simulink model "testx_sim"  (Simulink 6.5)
settings: Solver=ode45  StartTime=0.0  StopTime=300.0  RelTol=1e-3
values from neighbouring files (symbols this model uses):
  A = [ -0.195 0.195; 0.195 -0.205]    [testx.m]    (also in podklad.m = [dh1_h10 dh1_h20 0; kockaLQG.m = [0 1 0 0 0; kockaLQR.m = [0 1 0 0 0; kulicka_na_tyci_LQG_podklad.m = [0 0;1 0])
  B = [0.0047; 0]    [testx.m]    (also in podklad.m = [dh1_q0; kockaLQG.m = [0; kockaLQR.m = [0; kulicka_na_tyci_LQG_podklad.m = [7.14;0])
  C = [0 1]    [testx.m]    (also in podklad.m = [0 0 1]; kockaLQG.m = [1 0 0 0 0]; kockaLQR.m = [1 0 0 0 0]; kulicka_na_tyci_LQG_podklad.m)
  D = [0]    [testx.m]    (also in podklad.m = 0; kockaLQG.m; kockaLQR.m; kulicka_na_tyci_LQG_podklad.m = 0)
  K = tf(num,den)    [phinf2.m]
  Ng = Nu + K*Nx    [lqr_kompenzace.m]    (also in testx.m = lqr_kompenzace(A,B,C,D,K); kockaLQG.m = lqr_kompenzace(A,B,C,D,K); kockaLQR.m = lqr_kompenzace(A,B,C,D,K); kulicka_na_tyci_LQG_podklad.m = lqr_kompenzace(A,B,C,D,K))
undefined symbols (not defined in the file or in its folder): KA, KB, KC, KD, L
libraries: simulink_extras x2

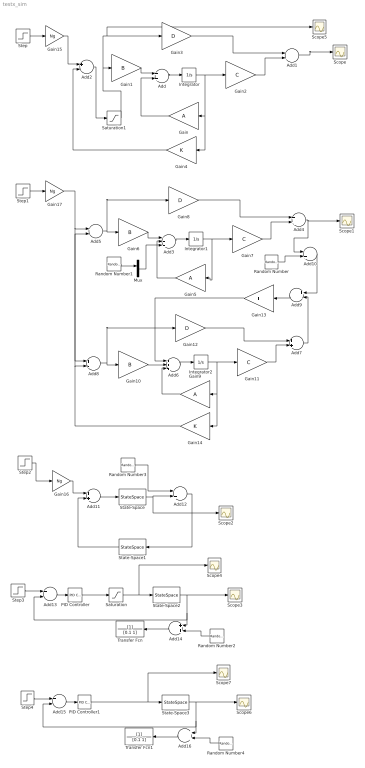
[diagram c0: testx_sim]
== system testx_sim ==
  Add{,1,4,7,10..12} (7 alike) : Sum  OutScaling=2^-10
  Add{2,5,8,13,15} (5 alike) : Sum  Inputs=+-  OutScaling=2^-10
  Add14 : Sum  Orientation=left  OutScaling=2^-10
  Add16 : Sum  Orientation=left  OutScaling=2^-10
  Add3 : Sum  Inputs=+++  OutScaling=2^-10
  Add6 : Sum  Inputs=+++  OutScaling=2^-10
  Add9 : Sum  Orientation=left  Inputs=+-  OutScaling=2^-10
  Gain : Gain  Orientation=left  Gain=A  Multiplication=Matrix(K*u) (u vector)
  Gain1 : Gain  Gain=B  Multiplication=Matrix(K*u) (u vector)
  Gain10 : Gain  Gain=B  Multiplication=Matrix(K*u) (u vector)
  Gain11 : Gain  Gain=C  Multiplication=Matrix(K*u) (u vector)
  Gain12 : Gain  Gain=D  Multiplication=Matrix(K*u) (u vector)
  Gain13 : Gain  Orientation=left  Gain=L  Multiplication=Matrix(K*u) (u vector)
  Gain14 : Gain  Orientation=left  Gain=K  Multiplication=Matrix(K*u) (u vector)
  Gain15 : Gain  Gain=Ng
  Gain16 : Gain  Gain=Ng
  Gain17 : Gain  Gain=Ng
  Gain2 : Gain  Gain=C  Multiplication=Matrix(K*u) (u vector)
  Gain3 : Gain  Gain=D  Multiplication=Matrix(K*u) (u vector)
  Gain4 : Gain  Orientation=left  Gain=K  Multiplication=Matrix(K*u) (u vector)
  Gain5 : Gain  Orientation=left  Gain=A  Multiplication=Matrix(K*u) (u vector)
  Gain6 : Gain  Gain=B  Multiplication=Matrix(K*u) (u vector)
  Gain7 : Gain  Gain=C  Multiplication=Matrix(K*u) (u vector)
  Gain8 : Gain  Gain=D  Multiplication=Matrix(K*u) (u vector)
  Gain9 : Gain  Orientation=left  Gain=A  Multiplication=Matrix(K*u) (u vector)
  Integrator : Integrator
  Integrator1 : Integrator
  Integrator2 : Integrator
  Mux : Mux  Inputs=2
  PID Controller : simulink_extras/Additional Linear/PID Controller  SystemSampleTime=-1  P=50  I=0.1  D=7
  PID Controller1 : simulink_extras/Additional Linear/PID Controller  SystemSampleTime=-1  P=500000  I=0.1  D=700000
  Random Number : RandomNumber  Variance=0  SampleTime=0
  Random Number1 : RandomNumber  Variance=0.002  SampleTime=0
  Random Number2 : RandomNumber  Orientation=left  Variance=0.00002  SampleTime=0
  Random Number3 : RandomNumber  Variance=0.02  SampleTime=0
  Random Number4 : RandomNumber  Orientation=left  Variance=0.00002  SampleTime=0
  Saturation : Saturate  UpperLimit=10  LowerLimit=0.0
  Saturation1 : Saturate  UpperLimit=10  LowerLimit=0.0
  Scope{,1..7} (8 alike) : Scope
  State-Space : StateSpace  A=A  B=B  C=C  D=D
  State-Space1 : StateSpace  Orientation=left  A=KA  B=KB  C=KC  D=KD
  State-Space2 : StateSpace  A=A  B=B  C=C  D=D
  State-Space3 : StateSpace  A=A  B=B  C=C  D=D
  Step{,1..4} (5 alike) : Step  Time=0  SampleTime=0
  Transfer Fcn : TransferFcn  Orientation=left  Denominator=[0.1 1]
  Transfer Fcn1 : TransferFcn  Orientation=left  Denominator=[0.1 1]
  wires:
  Gain1/1 -> Add/1
  Add/1 -> Integrator/1
  Integrator/1 -> Gain2/1, Gain/1, Gain4/1
  Add1/1 -> Scope/1
  Gain2/1 -> Add1/2
  Gain3/1 -> Add1/1
  Gain/1 -> Add/2
  Gain4/1 -> Add2/2
  Gain6/1 -> Add3/1
  Add3/1 -> Integrator1/1
  Integrator1/1 -> Gain7/1, Gain5/1
  Add4/1 -> Add10/1, Scope1/1
  Gain7/1 -> Add4/2
  Gain8/1 -> Add4/1
  Gain5/1 -> Add3/2
  Add5/1 -> Gain6/1, Gain8/1
  Gain10/1 -> Add6/2
  Add6/1 -> Integrator2/1
  Integrator2/1 -> Gain11/1, Gain9/1, Gain14/1
  Add7/1 -> Add9/2
  Gain11/1 -> Add7/2
  Gain12/1 -> Add7/1
  Gain9/1 -> Add6/3
  Random Number/1 -> Add10/2
  Add10/1 -> Add9/1
  Add9/1 -> Gain13/1
  Add8/1 -> Gain10/1, Gain12/1
  Gain14/1 -> Add8/2, Add5/2
  Mux/1 -> Add3/3
  Gain13/1 -> Add6/1
  Step3/1 -> Add13/1
  Add13/1 -> PID Controller/1
  State-Space2/1 -> Scope3/1, Add14/1, Add13/2
  Random Number2/1 -> Add14/2
  Add14/1 -> Transfer Fcn/1
  Add11/1 -> State-Space/1
  State-Space/1 -> Add12/2, Scope2/1
  Add12/1 -> State-Space1/1
  Random Number3/1 -> Add12/1
  State-Space1/1 -> Add11/2
  PID Controller/1 -> Saturation/1
  Saturation/1 -> State-Space2/1, Scope4/1
  Step/1 -> Gain15/1
  Gain15/1 -> Add2/1
  Gain16/1 -> Add11/1
  Step2/1 -> Gain16/1
  Step1/1 -> Gain17/1
  Gain17/1 -> Add8/1, Add5/1
  Random Number1/1 -> Mux/1
  Add2/1 -> Saturation1/1
  Saturation1/1 -> Gain1/1, Gain3/1, Scope5/1
  Step4/1 -> Add15/1
  Add15/1 -> PID Controller1/1
  State-Space3/1 -> Scope6/1, Add16/1, Add15/2
  Random Number4/1 -> Add16/2
  Add16/1 -> Transfer Fcn1/1
  PID Controller1/1 -> State-Space3/1, Scope7/1
